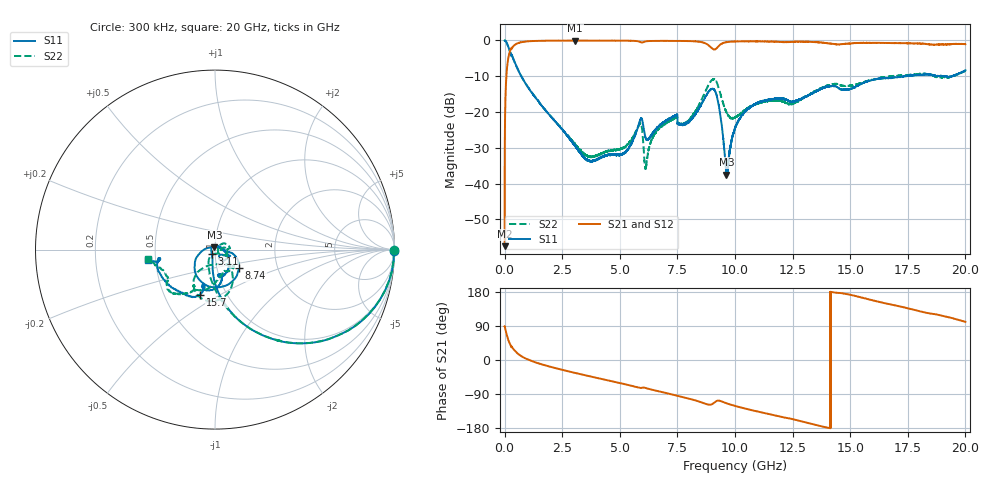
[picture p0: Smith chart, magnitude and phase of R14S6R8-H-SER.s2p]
!{R14S6R8}
!Johanson Technology Inc.
!www.johansontechnology.com
!Test Board Conditions:
!Substrate Type  RO4350B
!Substrate Thickness  20 mil
!Substrate Dk  3.66
!TL Type: GCPW
!TL Trace Width  36 mil
!TL Gap  12 mil
!Electrode orientation  Horizontal
!DUT TOPOLOGY	SERIES
!Mounting Pad LxW  26x36 mil
! Created Wed Nov 25 17:33:21 2020
! 2 Port Network Data from SP1.SP block
! freq  magS11  angS11  magS21  angS21  magS12  angS12  magS22  angS22
# khz S ma R 50
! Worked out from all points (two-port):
!   20001 points, 300 kHz to 20 GHz, reference 50 ohm
!   highest |S21| = -0.03 dB at 3.064 GHz (marker M1); lowest = -57.5 dB at 300 kHz (marker M2)
!   |S21| within 3 dB of the highest: 231.1 MHz to end of sweep
!   lowest |S11| = -37.4 dB at 9.623 GHz (marker M3), VSWR 1.03, Z = 49.7 + j1.3 ohm
!   |S11| at or under -10 dB: 725.6 MHz to 17.35 GHz (16.62 GHz wide, 184 % of centre); 19.1 GHz to 19.41 GHz (309.4 MHz wide, 1.61 % of centre); 19.41447 GHz to 19.41927 GHz (4.798 MHz wide, 0.0247 % of centre)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
!   |S22| runs from -35.9 to 0.0 dB; largest |S21 - S12| = 0.021
!   S11 on the Smith chart (normalised r, x): 300 kHz: open; 3.11 GHz: 0.96, -0.05; 8.74 GHz: 1.28, -0.27; 15.7 GHz: 0.75, -0.41; 20 GHz: 0.45, -0.06
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300  0.996 -0.3  0.001341 89.1  0.001332 88.5  0.9971 -0.2
110300  0.9005 -27.1  0.4311 62.8  0.4322 62.7  0.9006 -27.0
290300  0.6184 -55.2  0.78 34.5  0.7807 34.5  0.6189 -55.0
995300  0.227 -86.5  0.9713 1.7  0.9709 1.7  0.2278 -89.1
3064300  0.03336 -122.2  0.9963 -34.1  0.9955 -34.1  0.03533 -120.3
3110300  0.03162 -124.7  0.995 -34.8  0.9955 -34.8  0.03398 -119.0
3334300  0.02563 -140.1  0.9948 -38.0  0.9948 -37.9  0.02819 -109.6
5173300  0.02659 53.8  0.9928 -63.3  0.9915 -63.2  0.03216 -5.0
5869300  0.07547 -22.3  0.9571 -73.7  0.9564 -73.7  0.06862 -3.7
6144300  0.04185 -55.9  0.9744 -74.3  0.9747 -74.3  0.01761 17.2
6667300  0.06234 -31.6  0.9884 -82.3  0.9872 -82.3  0.05735 36.8
7399300  0.08934 -23.6  0.9841 -92.8  0.9839 -92.8  0.08186 9.8
7931300  0.07078 -12.8  0.9808 -100.8  0.9808 -100.8  0.07275 -23.0
8740300  0.1685 -37.8  0.9032 -116.0  0.9019 -116.0  0.202 -60.7
9192300  0.1761 -126.4  0.7718 -108.4  0.7735 -108.6  0.267 -112.6
9623300  0.01343 103.9  0.9459 -114.0  0.946 -114.1  0.1004 -114.9
1.00003e7  0.05924 -13.6  0.9677 -121.1  0.9671 -121.2  0.08377 -75.5
1.09943e7  0.1339 -58.2  0.9697 -136.1  0.97 -136.1  0.1321 -41.0
1.33343e7  0.1824 -79.0  0.9548 -168.7  0.9565 -168.7  0.1839 -89.5
1.57003e7  0.2645 -108.5  0.9271 161.7  0.9284 161.6  0.2672 -119.0
1.66673e7  0.2958 -123.2  0.9211 147.8  0.9132 147.5  0.3158 -128.0
2e7  0.3815 -171.1  0.8884 100.8  0.8884 101.1  0.3749 -172.4
